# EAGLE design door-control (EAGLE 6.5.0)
AUTHOR: Pat Pannuto; REV: 2; TITLE: RPi Door Control
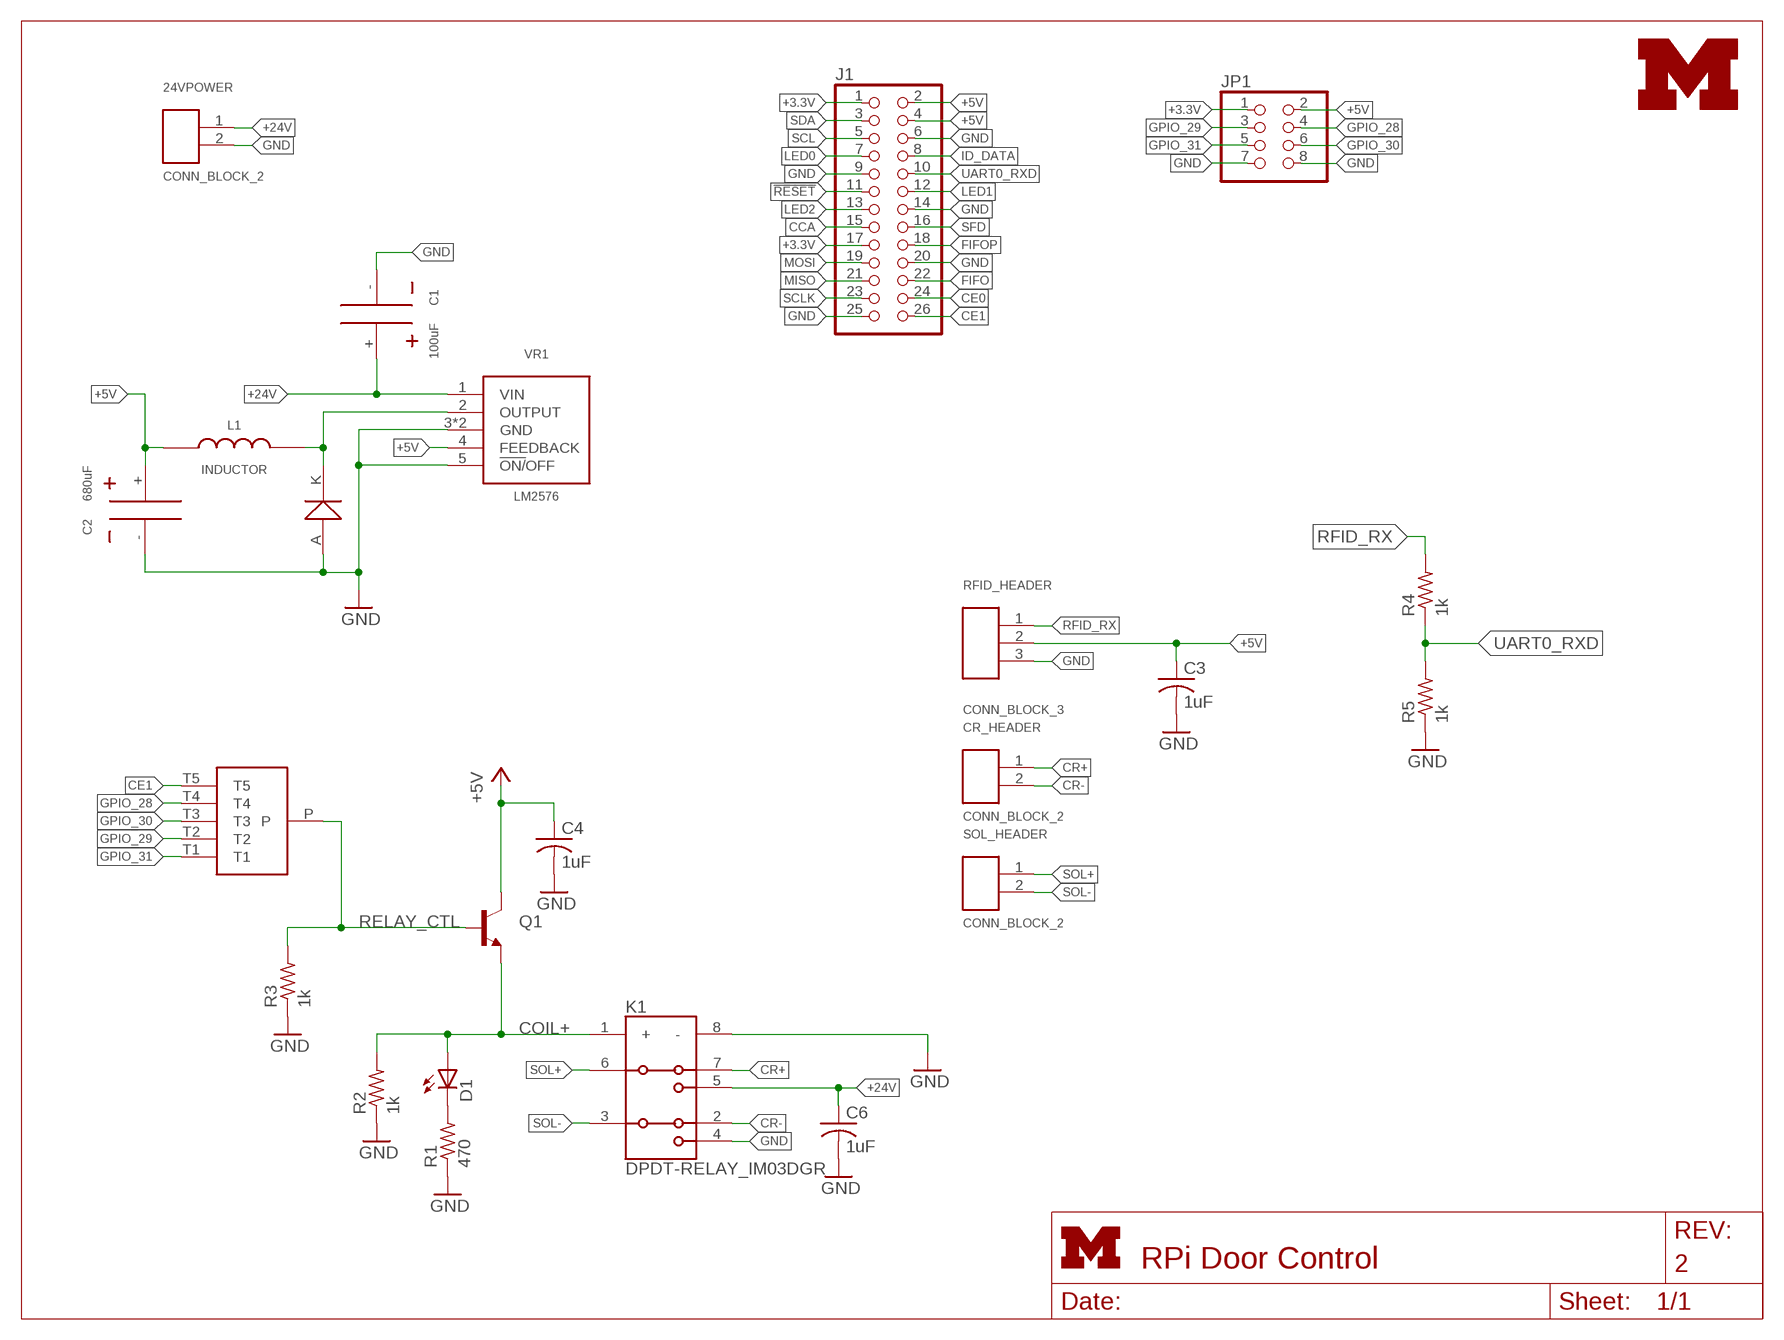
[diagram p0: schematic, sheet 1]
FRAME1 (LETTER_L): HEIGHT: 8.5in; WIDTH: 11in

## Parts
24VPOWER  CONN_BLOCK_2  [CONN_BLOCK_2]
C1  100uF  SMD_CAP_8MM_DIA  [SMD_CAP_8MM_DIA]
C2  680uF  SMD_CAP_8MM_DIA  [SMD_CAP_8MM_DIA]
C3  1uF  C-USC0603  [C0603]
C4  1uF  C-USC0603  [C0603]
C6  1uF  C-USC0603  [C0603]
CR_HEADER  CONN_BLOCK_2  [CONN_BLOCK_2]
D1  LED0603  [LED-0603]
D2  SMD_DIODE  [SMC_DIODE]
J1  PINHD-2X13  [2X13]
JP1  PINHD-2X4  [2X04]
K1  DPDT-RELAY_IM03DGR  [TE-DPDT-RELAY]
L1  INDUCTOR  [KM-5.0]
Q1  TRANSISTOR_NPNSOT23  [SOT23]
R1  470  R-US_R0603  [R0603]
R2  1k  R-US_R0603  [R0603]
R3  1k  R-US_R0603  [R0603]
R4  1k  R-US_R0603  [R0603]
R5  1k  R-US_R0603  [R0603]
RFID_HEADER  CONN_BLOCK_3  [CONN_BLOCK_3]
S1  SP5T_RESISTORS  [SP5T_0603_RESISTORS]
SOL_HEADER  CONN_BLOCK_2  [CONN_BLOCK_2]
U$1  UMICH_SOLID_SMALL  [UMICH_SOLID_75MIL]
VR1  LM2576  [D2PAKD2T]

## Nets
!RESET: J1.11
+3.3V: J1.1 J1.17 JP1.1
+5V: C2.+ C3.1 C4.1 J1.2 J1.4 JP1.2 L1.1 Q1.3(C) RFID_HEADER.2 VR1.4(FEEDBACK)
+24V: 24VPOWER.1 C1.+ C6.1 K1.5(Z1) VR1.1(VIN)
CCA: J1.15
CE0: J1.24
CE1: J1.26 S1.T5
COIL+: D1.A K1.1(+) Q1.2(E) R2.2
CR+: CR_HEADER.1 K1.7(Y1)
CR-: CR_HEADER.2 K1.2(Y2)
FIFO: J1.22
FIFOP: J1.18
GND: 24VPOWER.2 C1.- C2.- C3.2 C4.2 C6.2 D2.A J1.6 J1.9 J1.14 J1.20 J1.25 JP1.7 JP1.8 K1.4(Z2) K1.8(-) R1.1 R2.1 R3.1 R5.1 RFID_HEADER.3 VR1.3(GND) VR1.5(!ON/!OFF) VR1.PAD(GND)
GPIO_28: JP1.4 S1.T4
GPIO_29: JP1.3 S1.T2
GPIO_30: JP1.6 S1.T3
GPIO_31: JP1.5 S1.T1
ID_DATA: J1.8
LED0: J1.7
LED1: J1.12
LED2: J1.13
MISO: J1.21
MOSI: J1.19
N$1: D1.C R1.2
RELAY_CTL: Q1.1(B) R3.2 S1.P
RFID_RX: R4.2 RFID_HEADER.1
SCL: J1.5
SCLK: J1.23
SDA: J1.3
SFD: J1.16
SOL+: K1.6(A1) SOL_HEADER.1
SOL-: K1.3(A2) SOL_HEADER.2
UART0_RXD: J1.10 R4.1 R5.2
VREG_OUT: D2.K L1.2 VR1.2(OUTPUT)

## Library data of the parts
24VPOWER CR_HEADER SOL_HEADER = door-control:CONN_BLOCK_2: 2x 0.100 in screw terminal block; DIGIKEY: 277-1273-ND
C1 C2 = door-control:SMD_CAP_8MM_DIA; DIGIKEY: PCE4442CT-ND
C3 C4 C6 = resistor:C-US: CAPACITOR, American symbol
D1 = SparkFun-LED:LED: LEDs; DIGIKEY: 160-1834-1-ND
D2 = door-control:SMD_DIODE; DIGIKEY: MURS320-13FDICT-ND
J1 = pinhead:PINHD-2X13: PIN HEADER; DIGIKEY: SAM1204-13-ND
JP1 = pinhead:PINHD-2X4: PIN HEADER
K1 = door-control:DPDT-RELAY_IM03DGR; DIGIKEY: PB1172CT-ND
L1 = door-control:INDUCTOR: Inductor; DIGIKEY: 553-1574-5-ND
Q1 = door-control:TRANSISTOR_NPN: Transistor NPN BJT configuration in SOT23 package. MMBT2222 is the common NPN we use. Double check BCE configuration again layout.
R1-R5 = resistor:R-US_: RESISTOR, American symbol
RFID_HEADER = door-control:CONN_BLOCK_3: 3x 0.100 in screw terminal block; DIGIKEY: 277-1274-ND
S1 = door-control:SP5T_RESISTORS
U$1 = logos:UMICH_SOLID
VR1 = door-control:LM2576: Fixed Output Voltage Buck Regulator; DIGIKEY: LM2576D2T-005GOS-ND

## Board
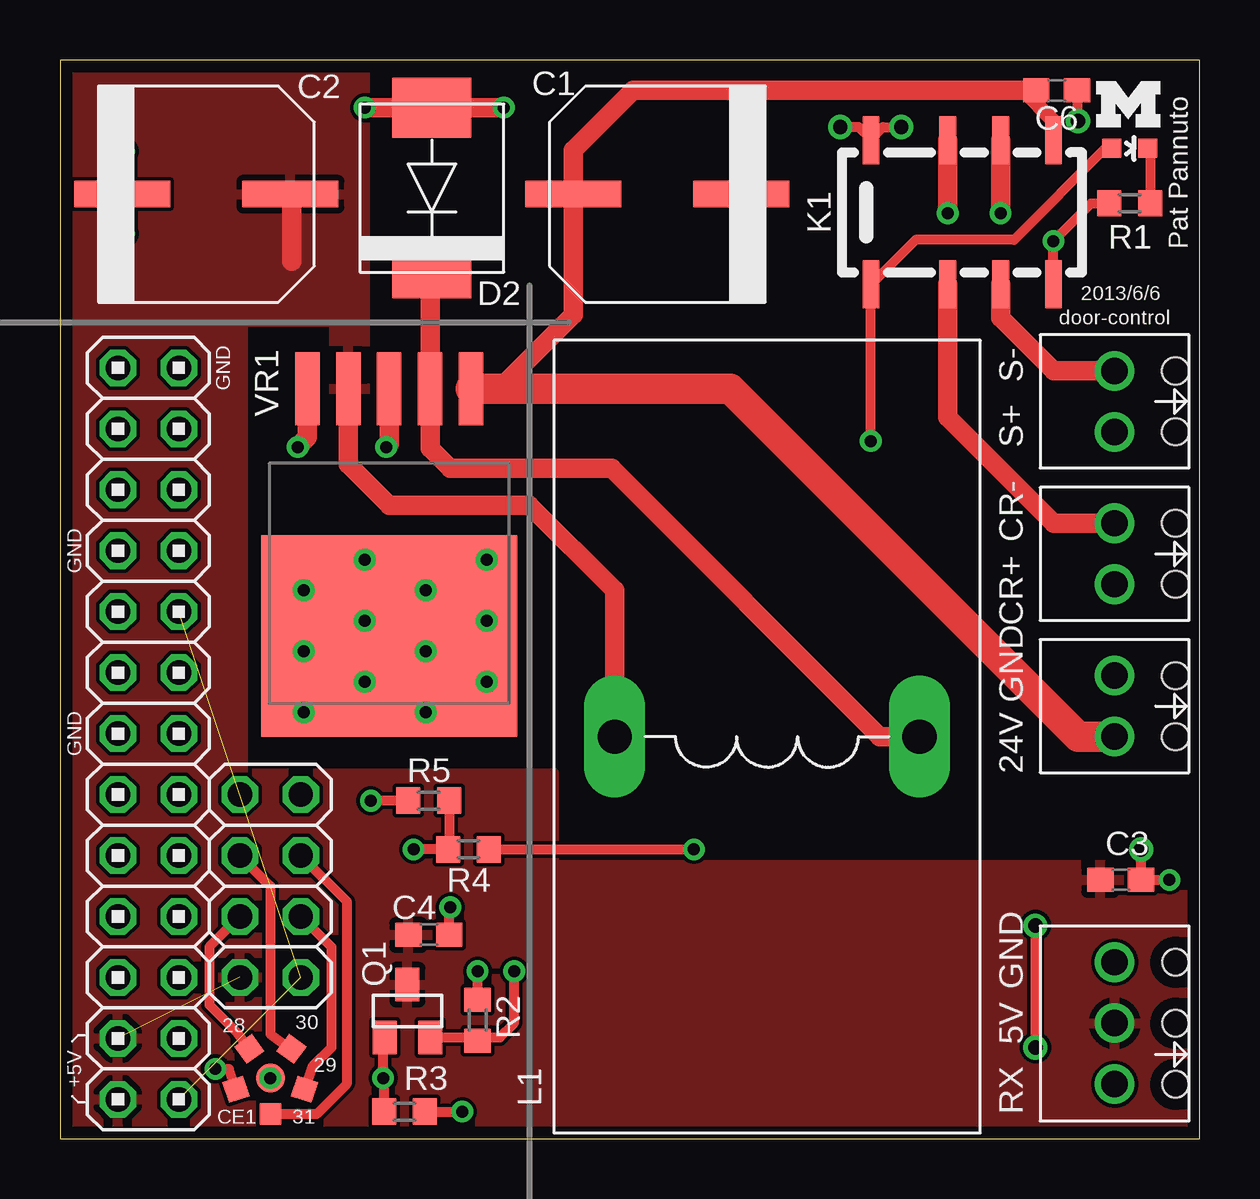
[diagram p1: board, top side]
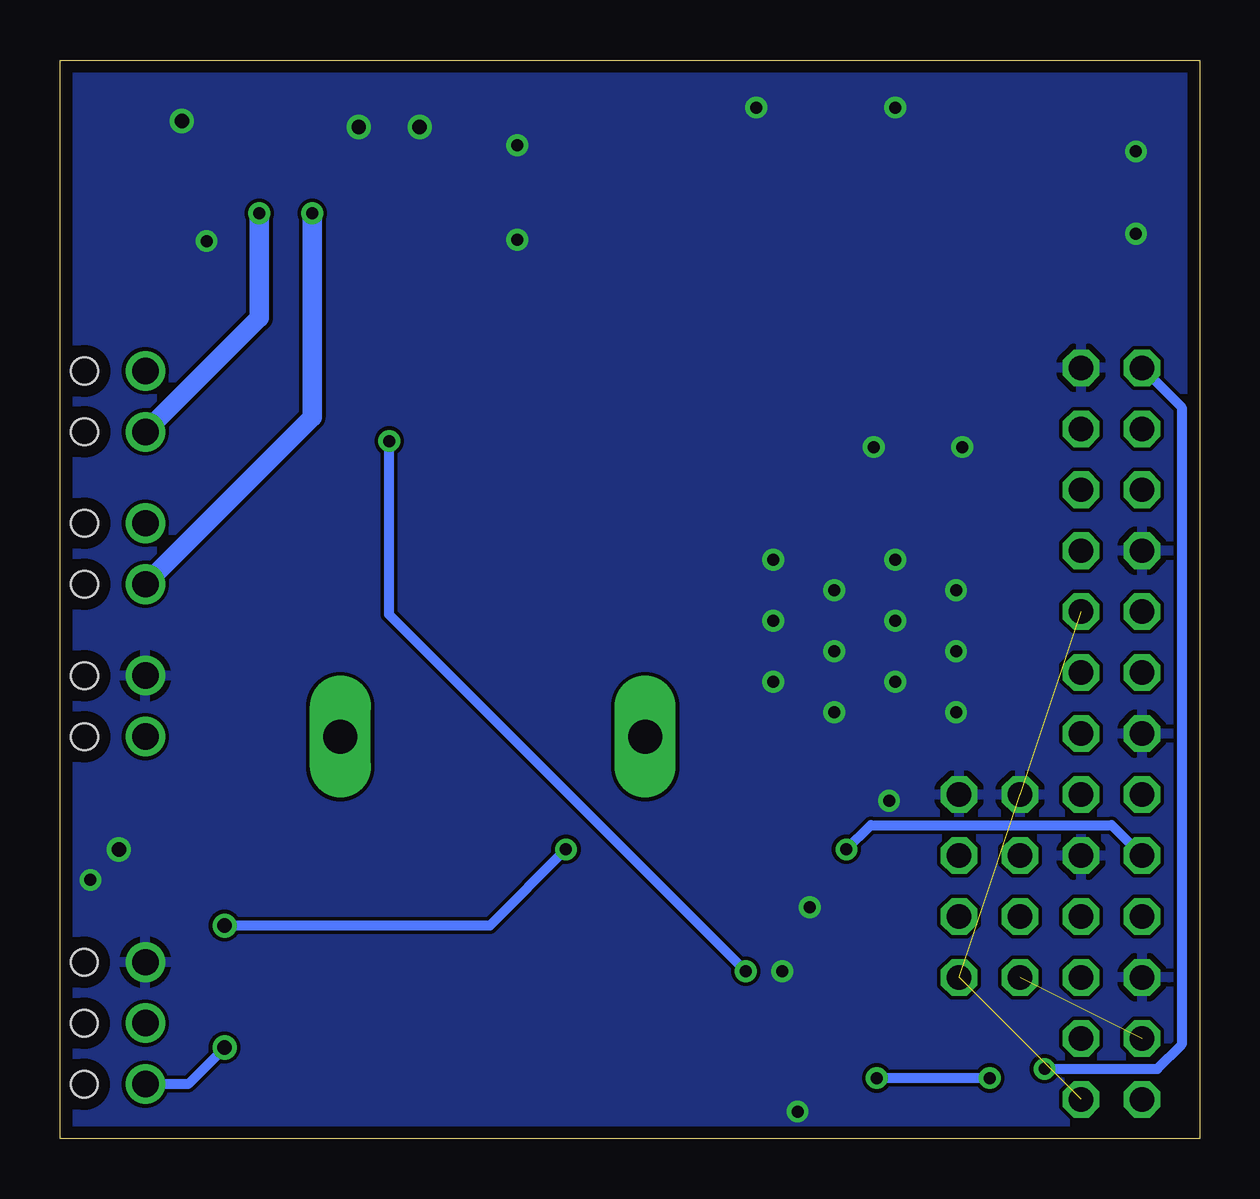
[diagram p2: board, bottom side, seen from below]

Size 47.5 x 44.96 mm. Coordinates in mm from the lower left corner, seen from the top.
Outline: 0,0 47.5,0 47.5,44.96 0,44.96 0,0
Copper layers (1*16): Top 0.0178mm / dielectric 59mil / Bottom 0.0178mm
Design rules "sunstone-2lyr_v1.0.0.3": minimum track width 6mil, minimum drill 14mil, track to track 6mil, track to pad 6mil, pad to pad 6mil, via to via 6mil, smd to smd 6mil, copper to edge 20mil, drill to drill 16mil, minimum pad ring 8mil, minimum via ring 8mil, stop-mask expansion 3mil, vias tented up to drill 0mil, thermal gap 10mil

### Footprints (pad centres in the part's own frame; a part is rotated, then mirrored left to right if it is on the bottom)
CONN_BLOCK_2 = drill 1.1: 1 -1.27,0; 2 1.27,0 | hole 1.12: -1.27,-2.54; 1.27,-2.54
SMD_CAP_8MM_DIA = smd 4 x 1.1: + 3.5,0; - -3.5,0
C0603 = smd 1.1 x 1: 1 -0.85,0; 2 0.85,0
LED-0603 = smd 0.8 x 0.8: A 0,-0.75; C 0,0.75
SMC_DIODE = smd 2.5 x 3.3: A 3.35,0; K -3.35,0
2X13 = drill 1.016 octagon: 1 -15.24,-1.27; 2 -15.24,1.27; 3 -12.7,-1.27; 4 -12.7,1.27; 5 -10.16,-1.27; 6 -10.16,1.27; 7 -7.62,-1.27; 8 -7.62,1.27; 9 -5.08,-1.27; 10 -5.08,1.27; 11 -2.54,-1.27; 12 -2.54,1.27; 13 0,-1.27; 14 0,1.27; 15 2.54,-1.27; 16 2.54,1.27; 17 5.08,-1.27; 18 5.08,1.27; 19 7.62,-1.27; 20 7.62,1.27; 21 10.16,-1.27; 22 10.16,1.27; 23 12.7,-1.27; 24 12.7,1.27; 25 15.24,-1.27; 26 15.24,1.27
2X04 = drill 1.016 octagon: 1 -3.81,-1.27; 2 -3.81,1.27; 3 -1.27,-1.27; 4 -1.27,1.27; 5 1.27,-1.27; 6 1.27,1.27; 7 3.81,-1.27; 8 3.81,1.27
TE-DPDT-RELAY = smd 0.7 x 2: 1 -3.8,-3; 2 -0.6,-3; 3 1.6,-3; 4 3.8,-3; 5 3.8,3; 6 1.6,3; 7 -0.6,3; 8 -3.8,3
KM-5.0 = drill 1.422 pad 2.54 long: 1 0,6.35; 2 0,-6.35
SOT23 = smd 1 x 1.4: 1 -0.95,-1.1; 2 0.95,-1.1; 3 0,1.1
R0603 = smd 1 x 1.1: 1 -0.85,0; 2 0.85,0
CONN_BLOCK_3 = drill 1.1: 1 -2.54,0; 2 0,0; 3 2.54,0 | hole 1.1: -2.54,-2.54; 0,-2.54; 2.54,-2.54
SP5T_0603_RESISTORS = smd 1.2 x 1.2: P 0,0 | smd 0.9 x 0.9: T1 1.5,0 | smd 0.9 x 0.9 rotated 72: T2 0.464,1.427 | smd 0.9 x 0.9 rotated 144: T3 -1.214,0.882 | smd 0.9 x 0.9 rotated 216: T4 -1.214,-0.882 | smd 0.9 x 0.9 rotated 288: T5 0.464,-1.427
D2PAKD2T = smd 3.05 x 1.016: 1 6.115,-3.404; 2 6.115,-1.702; 3 6.115,0; 4 6.115,1.702; 5 6.115,3.404 | smd 8.38 x 10.66: PAD -4.19,0

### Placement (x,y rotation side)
24VPOWER  43.94,18.03 90 top
C1  24.89,39.37 180 top
C2  6.1,39.37 0 top
C3  44.2,10.79 0 top
C4  15.37,8.51 0 top
C6  41.53,43.69 0 top
CR_HEADER  43.94,24.38 90 top
D1  44.58,41.27 270 top
D2  15.49,39.62 90 top
J1  3.68,16.89 90 top
JP1  8.76,10.54 90 top
K1  37.59,38.61 0 top
L1  29.46,16.76 90 top
Q1  14.48,5.33 0 top
R1  44.58,38.99 0 top
R2  17.4,4.95 270 top
R3  14.35,1.14 180 top
R4  17.02,12.06 0 top
R5  15.37,14.1 0 top
RFID_HEADER  43.94,4.83 90 top
S1  8.76,2.54 270 top
SOL_HEADER  43.94,30.73 90 top
U$1  43.18,42.16 0 top
VR1  13.72,25.15 90 top

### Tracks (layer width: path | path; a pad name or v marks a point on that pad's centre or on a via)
+3.3V  (2 unrouted)
+5V  (1 unrouted)
  Top 0.813: C2.+ 9.65,39.37 9.65,36.58 | L1.1 23.11,22.86 19.56,26.42 13.72,26.42 12.01,28.12 VR1.4
  pour Top: 0,44.96 12.7,44.96 12.7,29.84 11.43,29.84 11.43,34.04 7.62,34.04 7.62,15.24 20.57,15.24 20.57,11.43 47.5,11.43 47.5,0 0,0
+24V
  Top 0.406: C6.1 39.88,43.69
  Top 0.61: K1.5 41.39,42.43 40.13,43.69
  Top 0.813: VR1.1 18.31,31.26 21.39,34.35 C1.+ 21.39,41.2 23.88,43.69 39.88,43.69 40.13,43.69
  Top 1.27: VR1.1 27.92,31.26 42.42,16.76 24VPOWER.1
CE1  (via drill 0.5)
  Top 0.406: v6.48,2.92 7.04,2.92 S1.T5
  Bottom 0.406: J1.26 0.76,30.48 0.76,3.94 1.78,2.92 v6.48,2.92
COIL+  (via drill 0.5)
  Top 0.406: Q1.2 17.27,4.23 | 17.27,4.23 R2.2 | 17.27,4.23 18.33,4.23 18.92,4.83 v18.92,6.99 | D1.A 43.56,41.27 39.75,37.47 35.65,37.47 K1.1 33.78,35.6 v33.78,29.08
  Bottom 0.406: v18.92,6.99 33.78,21.84 v33.78,29.08
CR+  (via drill 0.5)
  Top 0.813: K1.7 v36.99,38.57
  Bottom 0.813: v36.99,38.57 36.99,30.06 CR_HEADER.1
CR-
  Top 0.813: K1.2 36.99,30.06 41.4,25.65 CR_HEADER.2
GND  (via drill 0.5, 0.6)
  Top 0.406: R3.1 v16.76,1.14 | R2.1 v17.4,6.99 | R5.1 v12.95,14.1 | C4.2 16.22,9.87 v16.26,9.65 | VR1.PAD 13.33,20.96 v12.7,21.59 | K1.4 v41.39,37.42 42.97,38.99 R1.1 | v46.23,10.79 C3.2 45.05,11.85 v45.05,12.06 | C6.2 42.38,42.71 v42.42,42.42 | v35.05,42.16 34.29,42.16 33.79,41.67 K1.8 33.79,41.65 33.27,42.16 v32.51,42.16
  Top 0.813: v18.49,42.98 v18.49,42.97 D2.A v12.7,42.97 v12.7,42.98 | C2.- 2.67,39.37 | 2.67,39.37 v2.67,41.15 | 2.67,39.37 v2.67,37.72 | v28.45,41.4 28.45,39.37 C1.- 28.39,37.47 v28.45,37.47 | VR1.5 10.31,29.23 v9.91,28.83 | VR1.3 13.72,28.96 v13.59,28.83
  other vias: 10.16,22.86 10.16,20.32 10.16,17.78 12.7,19.05 12.7,24.13 15.24,22.86 15.24,20.32 15.24,17.78 17.78,19.05 17.78,21.59 17.78,24.13
  pour Bottom: 0,0 0,44.96 47.5,44.96 47.5,0
GPIO_28
  Top 0.406: JP1.4 6.22,8 6.22,5.59 7.37,4.45 S1.T4
GPIO_29
  Top 0.406: JP1.3 11.3,8 11.3,3.81 10.54,3.05 S1.T2
GPIO_30
  Top 0.406: JP1.6 8.76,10.54 8.76,4.37 9.58,3.75 S1.T3
GPIO_31
  Top 0.406: JP1.5 11.94,9.91 11.94,2.29 10.69,1.04 S1.T1
N$1
  Top 0.406: D1.C 45.43,41.17 R1.2
RELAY_CTL  (via drill 0.5)
  Top 0.406: Q1.1 13.46,4.17 v13.46,2.54 13.5,2.5 R3.2
  Bottom 0.406: S1.P v13.46,2.54
  other vias: 8.76,2.54
RFID_RX  (via drill 0.5, 0.6)
  Top 0.406: v40.64,8.89 v40.64,3.81 | R4.2 v26.42,12.06
  Bottom 0.406: RFID_HEADER.1 42.16,2.29 v40.64,3.81 | v26.42,12.06 29.59,8.89 v40.64,8.89
SOL+  (via drill 0.5)
  Top 0.813: K1.6 v39.19,38.57
  Bottom 0.813: v39.19,38.57 39.19,34.21 SOL_HEADER.1
SOL-
  Top 0.813: K1.3 39.19,34.21 41.4,32 SOL_HEADER.2
UART0_RXD  (via drill 0.5)
  Top 0.406: v14.73,12.06 R4.1 16.22,12.11 R5.2
  Bottom 0.406: J1.10 3.68,13.08 13.72,13.08 v14.73,12.06
VREG_OUT
  Top 0.813: D2.K 15.42,36.2 VR1.2 15.42,28.78 16.26,27.94 22.99,27.94 34.16,16.76 L1.2

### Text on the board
tPlace: Pat Pannuto | 2013/6/6 | door-control | GND | S- | S+ | CR- | GND | CR+ | GND | GND | 24V | GND | 30 | 5V | 28 | +5V | 29 | RX | CE1 | 31
tDocu: CC2520 Edge

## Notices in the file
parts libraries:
SparkFun-LED: Licensing: CC v3.0 Share-Alike You are welcome to use this library for commercial purposes.
